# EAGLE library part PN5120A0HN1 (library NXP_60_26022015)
Transmission module The PN512 is a highly integrated transceiver IC for contactless communication at 13.56 MHz. This transceiver IC utilizes an outstanding modulation and demodulation concept completely integrated for different kinds of contactless communication methods and protocols at 13.56 MHz. AAL Eindhoven MK
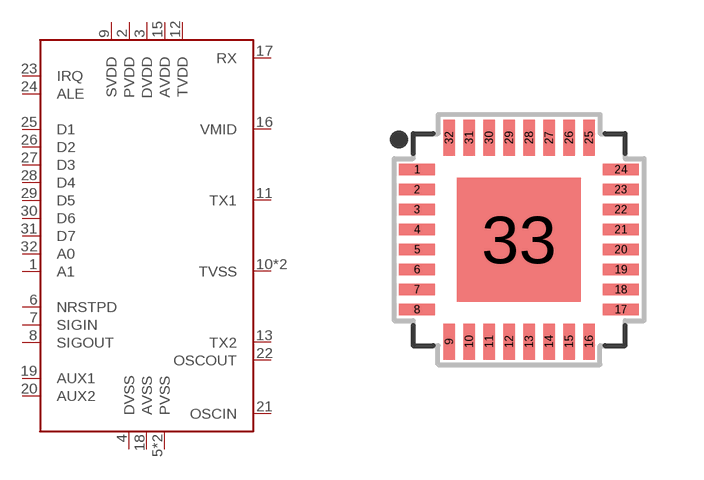
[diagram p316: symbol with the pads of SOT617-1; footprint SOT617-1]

Designator prefix U

## PN5120A0HN1  [SOT617-1]
1  A1  in
2  PVDD  pwr
3  DVDD  pwr
4  DVSS  pwr
5  PVSS  pwr
6  NRSTPD  in
7  SIGIN  in
8  SIGOUT  out
9  SVDD  pwr
10  TVSS
11  TX1
12  TVDD  pwr
13  TX2
14  TVSS
15  AVDD  pwr
16  VMID
17  RX
18  AVSS  pwr
19  AUX1  out
20  AUX2  out
21  OSCIN  in
22  OSCOUT  out
23  IRQ  out
24  ALE  in
25  D1
26  D2
27  D3
28  D4
29  D5
30  D6
31  D7
32  A0  in
33  PVSS  pwr

## Footprint SOT617-1 (pad centres in mm)
SOT617-1 HVQFN32: plastic thermal enhanced very thin quad flat package; no leads; 32 terminals; body 5 x 5 x 0.85 mm JEDEC: MO-220 IEC: ---
smd 0.9 x 0.29: 1 -2.55,1.75; 2 -2.55,1.25; 3 -2.55,0.75; 4 -2.55,0.25; 5 -2.55,-0.25; 6 -2.55,-0.75; 7 -2.55,-1.25; 8 -2.55,-1.75; 17 2.55,-1.75; 18 2.55,-1.25; 19 2.55,-0.75; 20 2.55,-0.25; 21 2.55,0.25; 22 2.55,0.75; 23 2.55,1.25; 24 2.55,1.75
smd 0.29 x 0.9: 9 -1.75,-2.55; 10 -1.25,-2.55; 11 -0.75,-2.55; 12 -0.25,-2.55; 13 0.25,-2.55; 14 0.75,-2.55; 15 1.25,-2.55; 16 1.75,-2.55; 25 1.75,2.55; 26 1.25,2.55; 27 0.75,2.55; 28 0.25,2.55; 29 -0.25,2.55; 30 -0.75,2.55; 31 -1.25,2.55; 32 -1.75,2.55
smd 3.1 x 3.1: 33 0,0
